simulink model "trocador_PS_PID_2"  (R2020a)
settings: Solver=VariableStepAuto  StartTime=0.0  StopTime=100  MaxStep=.01  RelTol=1e-3
libraries: cstblocks x6

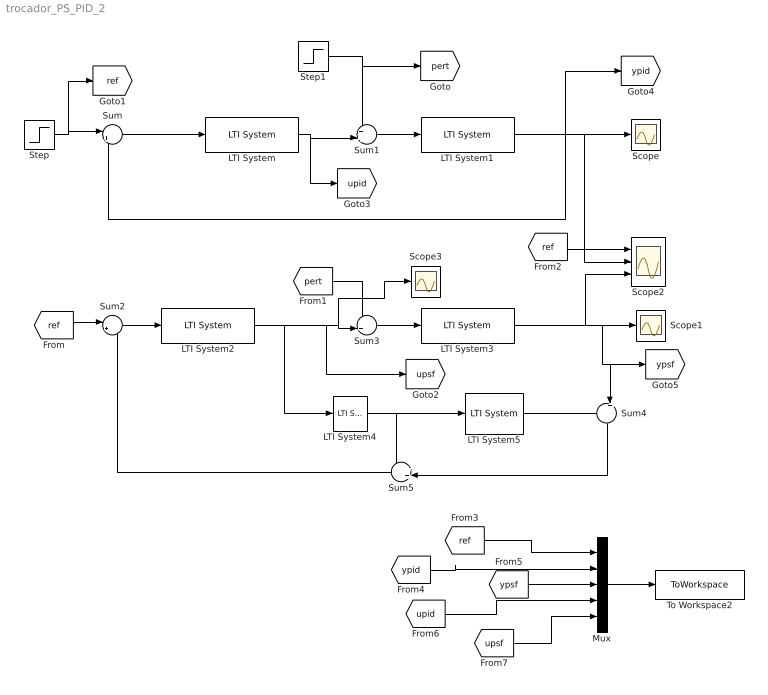
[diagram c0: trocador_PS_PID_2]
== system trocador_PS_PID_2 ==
  LTI System : cstblocks/LTI System  sys=C2z  IC=[]
  LTI System1 : cstblocks/LTI System  sys=P2  IC=[]
  LTI System2 : cstblocks/LTI System  sys=C1psz  IC=[]
  LTI System3 : cstblocks/LTI System  sys=P2  IC=[]
  LTI System4 : cstblocks/LTI System  sys=Gz  IC=[]
  LTI System5 : cstblocks/LTI System  sys=L2z  IC=[]
  Mux : Mux  Inputs=5
  Scope : Scope
  Scope1 : Scope
  Scope2 : Scope  NumInputPorts=3
  Scope3 : Scope
  Step : Step  Time=5  SampleTime=0
  Step1 : Step  Time=50  After=0.5  SampleTime=0
  Sum : Sum  Inputs=|+-
  Sum1 : Sum  Inputs=++|
  Sum2 : Sum  Inputs=|+-
  Sum3 : Sum  Inputs=++|
  Sum4 : Sum  Inputs=-+|
  Sum5 : Sum  Inputs=++|
  To Workspace2 : ToWorkspace  VariableName=simout  SampleTime=-1
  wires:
  Step/1 -> [ref], Sum/1
  Sum/1 -> LTI System/1
  LTI System/1 -> [upid], Sum1/2
  Step1/1 -> [pert], Sum1/1
  Sum1/1 -> LTI System1/1
  LTI System1/1 -> [ypid], Sum/2, Scope2/2, Scope/1
  Sum2/1 -> LTI System2/1
  [ref] -> Sum2/1
  LTI System2/1 -> [upsf], Scope3/1, Sum3/2, LTI System4/1
  Sum3/1 -> LTI System3/1
  LTI System3/1 -> Scope2/3, Scope1/1, [ypsf], Sum4/2
  [pert] -> Sum3/1
  LTI System4/1 -> Sum5/1, LTI System5/1
  LTI System5/1 -> Sum4/1
  Sum4/1 -> Sum5/2
  Sum5/1 -> Sum2/2
  [ref] -> Scope2/1
  Mux/1 -> To Workspace2/1
  [ref] -> Mux/1
  [ypid] -> Mux/2
  [ypsf] -> Mux/3
  [upid] -> Mux/4
  [upsf] -> Mux/5
